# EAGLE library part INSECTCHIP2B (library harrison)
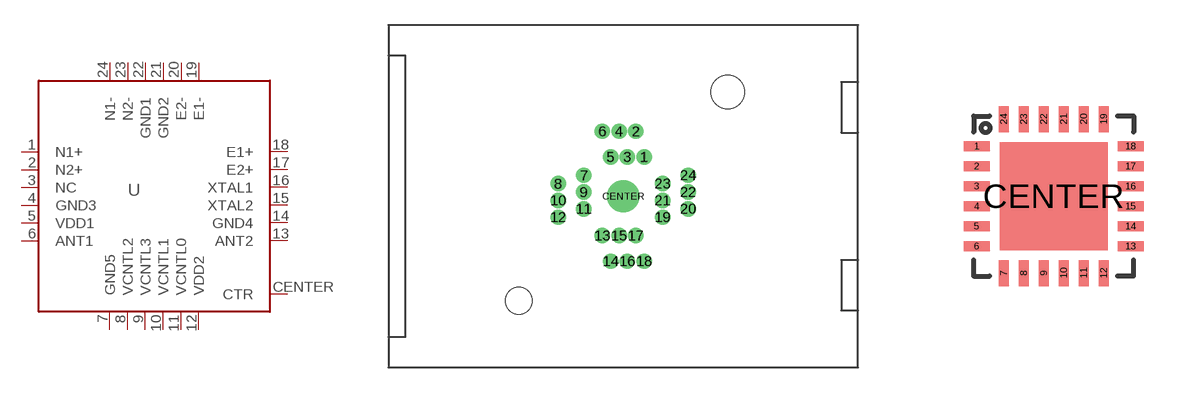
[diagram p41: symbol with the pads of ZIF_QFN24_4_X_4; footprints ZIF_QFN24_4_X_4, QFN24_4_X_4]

Designator prefix U

## INSECTCHIP2BZIF  [ZIF_QFN24_4_X_4]
1  N1+  in
2  N2+  in
3  NC  pas
4  GND3  pwr
5  VDD1  pwr
6  ANT1  pas
7  GND5  pwr
8  VCNTL2  in
9  VCNTL3  in
10  VCNTL1  in
11  VCNTL0  in
12  VDD2  pwr
13  ANT2  pas
14  GND4  pwr
15  XTAL2  pas
16  XTAL1  pas
17  E2+  in
18  E1+  in
19  E1-  in
20  E2-  in
21  GND2  pwr
22  GND1  pwr
23  N2-  in
24  N1-  in
CENTER  CTR  pwr

## INSECTCHIP2BQFN  [QFN24_4_X_4]
Pads as for ZIF_QFN24_4_X_4

## INSECTCHIP2BCOB  [INSECTCHIP2_COB]
Pads as for ZIF_QFN24_4_X_4

## Footprint ZIF_QFN24_4_X_4 (pad centres in mm)
drill 0.41 pad 0.813: 1 1.25,2.35; 2 0.75,3.875; 3 0.25,2.35; 4 -0.25,3.875; 5 -0.75,2.35; 6 -1.25,3.875; 7 -2.35,1.25; 8 -3.875,0.75; 9 -2.35,0.25; 10 -3.875,-0.25; 11 -2.35,-0.75; 12 -3.875,-1.25; 13 -1.25,-2.35; 14 -0.75,-3.875; 15 -0.25,-2.35; 16 0.25,-3.875; 17 0.75,-2.35; 18 1.25,-3.875; 19 2.35,-1.25; 20 3.875,-0.75; 21 2.35,-0.25; 22 3.875,0.25; 23 2.35,0.75; 24 3.875,1.25
drill 1.02 pad 1.93: CENTER 0,0
hole 1.6 at -6.23,-6.23
hole 2 at 6.22,6.22

## Footprint QFN24_4_X_4 (pad centres in mm)
smd 0.65 x 0.25: 1 -1.925,1.25; 2 -1.925,0.75; 3 -1.925,0.25; 4 -1.925,-0.25; 5 -1.925,-0.75; 6 -1.925,-1.25; 13 1.925,-1.25; 14 1.925,-0.75; 15 1.925,-0.25; 16 1.925,0.25; 17 1.925,0.75; 18 1.925,1.25
smd 0.25 x 0.65: 7 -1.25,-1.925; 8 -0.75,-1.925; 9 -0.25,-1.925; 10 0.25,-1.925; 11 0.75,-1.925; 12 1.25,-1.925; 19 1.25,1.925; 20 0.75,1.925; 21 0.25,1.925; 22 -0.25,1.925; 23 -0.75,1.925; 24 -1.25,1.925
smd 2.7 x 2.7: CENTER 0,0

## Footprint INSECTCHIP2_COB (pad centres in mm)
smd 0.254 x 0.254: 1 -1.714,1.27; 2 -1.714,0.762; 3 -1.714,0.254; 4 -1.714,-0.254; 5 -1.714,-0.762; 6 -1.714,-1.27; 7 -1.27,-1.714; 8 -0.762,-1.714; 9 -0.254,-1.714; 10 0.254,-1.714; 11 0.762,-1.714; 12 1.27,-1.714; 13 1.714,-1.27; 14 1.714,-0.762; 15 1.714,-0.254; 16 1.714,0.254; 17 1.714,0.762; 18 1.714,1.27; 19 1.27,1.714; 20 0.762,1.714; 21 0.254,1.714; 22 -0.254,1.714; 23 -0.762,1.714; 24 -1.27,1.714
smd 2.413 x 2.413: CENTER 0,0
